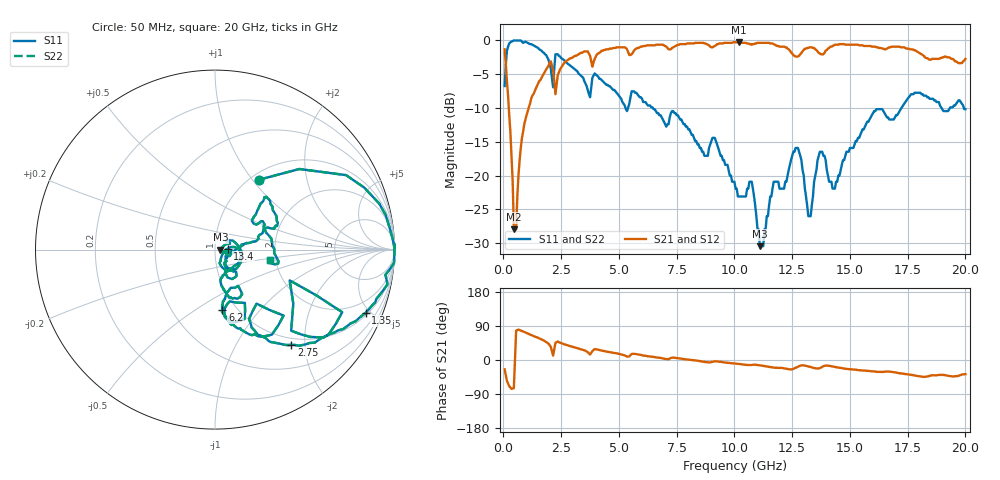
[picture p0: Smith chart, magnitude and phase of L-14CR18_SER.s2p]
# MHZ S MA R 50
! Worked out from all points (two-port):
!   400 points, 50 MHz to 20 GHz, reference 50 ohm
!   highest |S21| = -0.26 dB at 10.2 GHz (marker M1); lowest = -28.0 dB at 450 MHz (marker M2)
!   |S21| within 3 dB of the highest: 2.642 GHz to 3.811 GHz (1.169 GHz wide, 36.2 % of centre); 3.897 GHz to 19.67 GHz (15.77 GHz wide, 134 % of centre)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
!   lowest |S11| = -30.5 dB at 11.1 GHz (marker M3), VSWR 1.06, Z = 53.1 - j0.111 ohm
!   |S11| at or under -10 dB: 5.284 GHz to 5.391 GHz (106.7 MHz wide, 2 % of centre); 6.469 GHz to 17.23 GHz (10.76 GHz wide, 90.8 % of centre); 18.97 GHz to 19.33 GHz (362.6 MHz wide, 1.89 % of centre)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
!   |S22| runs from -30.5 to 0.0 dB; largest |S21 - S12| = 0
!   S11 on the Smith chart (normalised r, x): 50 MHz: 1.09, +1.08; 1.35 GHz: 1.14, -4.69; 2.75 GHz: 0.88, -1.73; 6.2 GHz: 0.86, -0.65; 13.4 GHz: 1.15, +0.01; 20 GHz: 1.86, -0.23
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50  0.46 57.8  0.86 -24.7  0.86 -24.7  0.46 57.8
200  0.9 22.6  0.39 -62.0  0.39 -62.0  0.9 22.6
450  1 0.5  0.04 -74.3  0.04 -74.3  1 0.5
800  0.98 -6.4  0.19 76.5  0.19 76.5  0.98 -6.4
1350  0.91 -22.8  0.42 61.8  0.42 61.8  0.91 -22.8
2150  0.45 -22.4  0.6 11.6  0.6 11.6  0.45 -22.4
2250  0.79 -26.2  0.4 45.3  0.4 45.3  0.79 -26.2
2750  0.68 -51.3  0.71 39.1  0.71 39.1  0.68 -51.3
3400  0.54 -62.3  0.81 27.9  0.81 27.9  0.54 -62.3
6200  0.34 -83.0  0.92 10.5  0.92 10.5  0.34 -83.0
6700  0.29 -80.2  0.93 6.3  0.93 6.3  0.29 -80.2
10050  0.08 -42.9  0.97 -9.4  0.97 -9.4  0.08 -42.9
10200  0.07 -29.7  0.97 -10.4  0.97 -10.4  0.07 -29.7
10750  0.09 -9.7  0.93 -13.1  0.93 -13.1  0.09 -9.7
11100  0.03 -2.0  0.96 -14.1  0.96 -14.1  0.03 -2.0
12650  0.16 -26.0  0.76 -20.6  0.76 -20.6  0.16 -26.0
13350  0.06 -1.0  0.89 -19.6  0.89 -19.6  0.06 -1.0
13400  0.07 4.1  0.88 -20.4  0.88 -20.4  0.07 4.1
13700  0.15 -12.6  0.8 -21.2  0.8 -21.2  0.15 -12.6
14350  0.08 -28.4  0.93 -18.2  0.93 -18.2  0.08 -28.4
16700  0.26 33.6  0.89 -30.7  0.89 -30.7  0.26 33.6
20000  0.31 -10.3  0.73 -37.5  0.73 -37.5  0.31 -10.3
